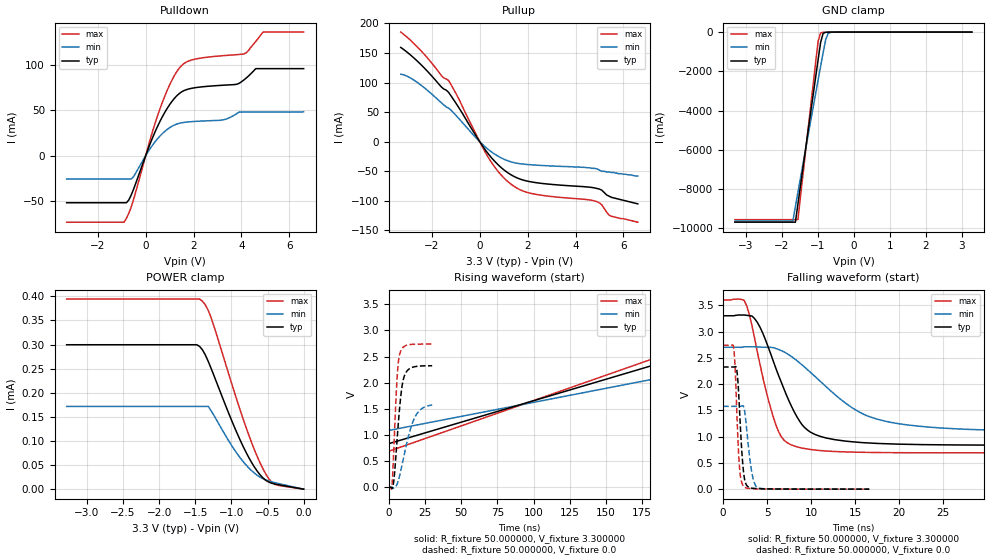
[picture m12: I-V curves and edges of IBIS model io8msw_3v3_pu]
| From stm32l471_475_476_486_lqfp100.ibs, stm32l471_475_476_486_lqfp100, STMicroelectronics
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|   Model io8msw_3v3_pu
[Model]  io8msw_3v3_pu
Model_type I/O
Polarity   Non-Inverting
Enable   Active-Low
Vinl =   0.990000V
Vinh =   2.310000V
Vmeas =  1.650000V
Cref =   100.000000nF
Rref =   1.000000k
Vref =   3.300000V
C_comp   2.968600pF   2.938100pF   3.196200pF
[Temperature Range]   25.000000   0.125000k   -40.000000
[Pullup Reference]   3.300000V   2.700000V   3.600000V
[Pulldown Reference]   0.0V   0.0V   0.0V
[POWER Clamp Reference]   3.300000V   2.700000V   3.600000V
[GND Clamp Reference]   0.0V   0.0V   0.0V
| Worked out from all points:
|   slope of the pulldown table from 0 to 0.495 V, typ, clamps not added: 15.4 ohm
|   slope of the pullup table from 0 to 0.495 V, typ, clamps not added: 18.1 ohm
|   GND clamp passes 1 mA (typ) near -0.58 V on its own axis
|   rising waveform, R_fixture 50.000000, V_fixture 3.300000: 20-80 % time 180ns typ, 180ns min, 180ns max; typ from 0.836 V to 3.3 V
|   rising waveform, R_fixture 50.000000, V_fixture 0.0: 20-80 % time 4.24ns typ, 8.5ns min, 2.78ns max; typ from 0.001 V to 2.33 V
|   falling waveform, R_fixture 50.000000, V_fixture 3.300000: 20-80 % time 3.67ns typ, 7.29ns min, 2.5ns max; typ from 3.3 V to 0.836 V
|   falling waveform, R_fixture 50.000000, V_fixture 0.0: 20-80 % time 486ps typ, 659ps min, 410ps max; typ from 2.33 V to 0.001 V
[Pulldown]
|Voltage   I(typ)   I(min)   I(max)
-3.3V     -51.62mA   -25.53mA   -73.04mA
-900mV    -51.62mA   -25.53mA   -73.04mA
-500mV    -36.51mA   -22.79mA   -47.71mA
200mV     14.02mA    8.316mA    18.9mA
700mV     42.98mA    24.4mA     58.9mA
1.2V      63.06mA    33.8mA     88.14mA
1.6V      71.63mA    36.67mA    101.4mA
3.2V      77.51mA    39.29mA    110mA
4.1V      83.28mA    47.99mA    112mA
4.6V      95.81mA    47.99mA    125.7mA
4.9V      95.81mA    47.99mA    136mA
6.6V      95.81mA    48.43mA    136mA
[Pullup]
|Voltage   I(typ)   I(min)   I(max)
-3.3V     159.4mA    114.2mA    185.3mA
-2.6V     136mA      99.99mA    159.9mA
-1.6V     92.47mA    65.73mA    111.7mA
-1.3V     83.33mA    56.75mA    103.4mA
300mV     -17.49mA   -11.19mA   -22.71mA
800mV     -40.27mA   -25.28mA   -51.87mA
1.3V      -55.74mA   -33.93mA   -71.59mA
2.2V      -68.23mA   -39.11mA   -87.81mA
4.8V      -78.1mA    -45mA      -100.2mA
5.1V      -82mA      -50mA      -106.7mA
5.5V      -94mA      -52mA      -126mA
6.6V      -105mA     -58mA      -136mA
[GND_clamp]
|Voltage   I(typ)   I(min)   I(max)
-3.3V     -9.687A    -9.633A    -9.557A
-1.69V    -9.687A    -9.633A    -9.557A
-1.62V    -9.687A    -8.894A    -9.557A
-1.55V    -8.764A    -8.167A    -9.557A
-1.13V    -3.236A    -3.867A    -2.713A
-990mV    -1.416A    -2.448A    -480.1mA
-920mV    -530mA     -1.746A    -39.96mA
-850mV    -62.36mA   -1.055A    -14.04mA
-780mV    -12.04mA   -390.4mA   -9.013mA
-710mV    -4.897mA   -69.08mA   -5.32mA
-640mV    -2.305mA   -14.59mA   -2.498mA
3.28V     0A         0A         0A
[POWER_clamp]
|Voltage   I(typ)   I(min)   I(max)
-3.28V    299.6uA    171.7uA    394.3uA
-1.48V    299.6uA    171.7uA    394.3uA
-1.4V     288.9uA    171.7uA    389.8uA
-1.32V    265uA      171.7uA    370.8uA
-1.28V    250.3uA    162.5uA    355.4uA
-1V       143.8uA    91.34uA    220.9uA
-840mV    89.44uA    57.68uA    146.9uA
-680mV    45.53uA    33.16uA    81.3uA
-560mV    22.92uA    21.5uA     41.26uA
-480mV    14.5uA     16.78uA    21.17uA
-400mV    10.75uA    13.5uA     10.02uA
0V        0A         5.458nA    0A
[Ramp]
| variable   typ   min   max
dV/dt_r  1.37848/4.14919n   0.74586/6.14058n   1.64102/2.77242n
dV/dt_f  1.45405/3.56485n   0.79458/5.42599n   1.74040/2.48283n
R_load = 50.000000
[Rising Waveform]
R_fixture= 50.000000
V_fixture= 3.300000
V_fixture_min= 2.700000
V_fixture_max= 3.600000
|time   V(typ)   V(min)   V(max)
0s        836mV      1.089V     690.6mV
300.3ns   3.3V       2.7V       3.6V
600.6ns   3.3V       2.7V       3.6V
29.73us   3.3V       2.7V       3.6V
[Rising Waveform]
R_fixture= 50.000000
V_fixture= 0.0
V_fixture_min= 0.0
V_fixture_max= 0.0
|time   V(typ)   V(min)   V(max)
0s        932.4uV    1.4mV      660.9uV
1.622ns   -1.432mV   1.4mV      -34.86mV
2.222ns   -16.42mV   1.582mV    70.65mV
3.544ns   163.6mV    -2.628mV   822.6mV
5.646ns   904.7mV    62.3mV     2.083V
7.447ns   1.531V     227.3mV    2.547V
9.489ns   2.002V     483.1mV    2.667V
12.19ns   2.214V     828.9mV    2.717V
19.28ns   2.313V     1.406V     2.737V
29.91ns   2.325V     1.576V     2.739V
[Falling Waveform]
R_fixture= 50.000000
V_fixture= 3.300000
V_fixture_min= 2.700000
V_fixture_max= 3.600000
|time   V(typ)   V(min)   V(max)
0s        3.3V       2.7V       3.6V
2.703ns   3.307V     2.711V     3.484V
4.204ns   3.082V     2.704V     2.374V
5.405ns   2.58V      2.699V     1.548V
6.607ns   2.042V     2.638V     1.003V
8.709ns   1.293V     2.403V     793.4mV
10.51ns   1.038V     2.136V     743.8mV
16.52ns   880.2mV    1.387V     700.1mV
27.03ns   841.6mV    1.145V     691.3mV
149.5ns   836mV      1.089V     690.6mV
[Falling Waveform]
R_fixture= 50.000000
V_fixture= 0.0
V_fixture_min= 0.0
V_fixture_max= 0.0
|time   V(typ)   V(min)   V(max)
0s        2.325V     1.576V     2.739V
1.201ns   2.325V     1.576V     2.696V
1.368ns   2.33V      1.576V     2.34V
1.568ns   2.264V     1.576V     1.471V
1.869ns   1.527V     1.576V     425.1mV
2.336ns   321.6mV    1.573V     54.89mV
2.636ns   87.31mV    1.228V     23.79mV
3.237ns   20.61mV    353.4mV    12.47mV
3.871ns   12.01mV    35.85mV    6.487mV
16.62ns   932.4uV    1.4mV      660.9uV
